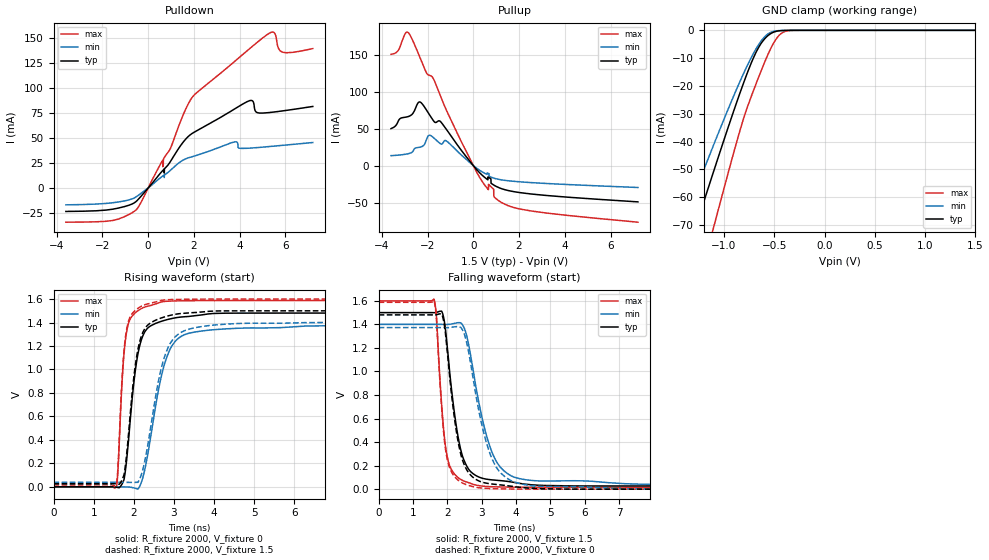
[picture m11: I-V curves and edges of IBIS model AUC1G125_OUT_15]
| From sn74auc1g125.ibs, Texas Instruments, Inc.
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[Model]   AUC1G125_OUT_15
Model_type  3-state
Enable   Active-Low
Vref =   0
Rref =   2000
Cref =   15p
Vmeas =   0.75
| variable   typ   min   max
C_comp   8.47pF   5.30pF   18.91pF
| C_pullup   7.46pF   4.00pF   14.06pF
| C_pulldown   10.53pF   5.76pF   20.41pF
| C_tri-state   8.47pF   5.30pF   18.91pF
[Temperature Range]   40   100   -40
| Ambient temperature   25   85   -40
[Voltage range]   1.5   1.4   1.6
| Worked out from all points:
|   slope of the pulldown table from 0 to 0.225 V, typ, clamps not added: 37 ohm
|   slope of the pullup table from 0 to 0.225 V, typ, clamps not added: 28.1 ohm
|   GND clamp passes 1 mA (typ) near -0.53 V on its own axis
|   rising waveform, R_fixture 2000, V_fixture 0: 20-80 % time 294ps typ, 469ps min, 169ps max; typ from 0 V to 1.48 V
|   falling waveform, R_fixture 2000, V_fixture 1.5: 20-80 % time 403ps typ, 622ps min, 244ps max; typ from 1.5 V to 0.027 V
|   rising waveform, R_fixture 2000, V_fixture 1.5: 20-80 % time 291ps typ, 461ps min, 167ps max; typ from 0.027 V to 1.5 V
|   falling waveform, R_fixture 2000, V_fixture 0: 20-80 % time 400ps typ, 617ps min, 242ps max; typ from 1.48 V to 0 V
[GND Clamp]
| AUC1G125_OUT_15A
|   Voltage   I(typ)   I(min)   I(max)
-3.6V     -338.8mA   -286.3mA   -409.7mA
-1.415V   -86.02mA   -70.29mA   -113.7mA
-1.265V   -68.97mA   -56.18mA   -93.1mA
-1.125V   -53.25mA   -43.26mA   -73.93mA
-1.085V   -48.8mA    -39.63mA   -68.47mA
-840mV    -22.47mA   -18.35mA   -35.96mA
-690mV    -8.595mA   -7.233mA   -20.12mA
-570mV    -2.132mA   -1.506mA   -9.318mA
-495mV    -520.9uA   -290.7uA   -3.905mA
-430mV    -104.6uA   -59.7uA    -1.117mA
-285mV    -1.435uA   -1.295uA   -9.372uA
1.5V      350.7pA    6.413nA    352.9pA
[Pulldown]
| AUC1G125_OUT_15A
|   Voltage   I(typ)   I(min)   I(max)
-3.6V     -23.47mA   -16.88mA   -34.23mA
-530mV    -13.56mA   -8.913mA   -21.94mA
630mV     17.27mA    11.79mA    27.62mA
655mV     17.88mA    12.18mA    21.8mA
1.92V     54.51mA    31.29mA    90.56mA
3.785V    79.13mA    46.19mA    126.7mA
4.44V     87.4mA     39.87mA    139.4mA
4.73V     75.86mA    40.35mA    145mA
5.195V    75.25mA    41.24mA    153.3mA
5.52V     76.05mA    41.91mA    155.3mA
5.885V    77.14mA    42.68mA    135.8mA
7.2V      81.56mA    45.48mA    139.5mA
[Pullup]
| AUC1G125_OUT_15A
|   Voltage   I(typ)   I(min)   I(max)
-3.6V     50.13mA    13.5mA     150.8mA
-2.81V    66.89mA    16.45mA    178.9mA
-2.355V   86.34mA    24.86mA    148.1mA
-1.89V    67.6mA     41.14mA    122.1mA
-1.415V   59mA       29.23mA    92.64mA
-1.175V   48.95mA    33.41mA    74.96mA
170mV     -6.178mA   -4.065mA   -10.23mA
890mV     -26.25mA   -16.87mA   -32.02mA
905mV     -26.53mA   -17.02mA   -41.95mA
1.12V     -29.9mA    -18.7mA    -47.79mA
2.525V    -38.43mA   -23mA      -61.43mA
7.2V      -49.13mA   -29.64mA   -76.65mA
[Ramp]
| AUC1G125_OUT_15A
| variable   typ   min   max
dV/dt_r   0.89/2.96E-10   0.84/4.79E-10   0.96/1.71E-10
dV/dt_f   0.89/4.06E-10   0.82/6.27E-10   0.96/2.46E-10
R_load = 2000
[Rising Waveform]
| AUC1G125_OUT_15A
R_fixture =   2000
C_fixture =   0
L_fixture =   0
V_fixture =   0
V_fixture_min = 0
V_fixture_max = 0
|   Time   V(typ)   V(min)   V(max)
0s        6.387nV    23.65nV    864.9pV
1.57ns    -3.297mV   8.561uV    4.787mV
1.735ns   43.44mV    -139.1uV   1.039V
1.855ns   343.3mV    -1.642mV   1.375V
2.015ns   925.7mV    -10.26mV   1.476V
2.165ns   1.225V     17.78mV    1.514V
2.73ns    1.415V     1.001V     1.578V
3.195ns   1.448V     1.285V     1.585V
4.585ns   1.48V      1.351V     1.587V
29.99ns   1.481V     1.373V     1.587V
[Falling Waveform]
| AUC1G125_OUT_15A
R_fixture =   2000
C_fixture =   0
L_fixture =   0
V_fixture =   1.5
V_fixture_min = 1.4
V_fixture_max = 1.6
|   Time   V(typ)   V(min)   V(max)
0s        1.5V       1.4V       1.6V
1.61ns    1.499V     1.4V       1.615V
1.68ns    1.502V     1.4V       1.474V
1.835ns   1.511V     1.4V       713.3mV
2.025ns   1.129V     1.399V     240mV
2.365ns   366.6mV    1.414V     87.16mV
2.89ns    106.6mV    777.3mV    31.27mV
3.465ns   74.44mV    217.1mV    19.05mV
4.455ns   36.93mV    73.69mV    16.52mV
29.99ns   27.18mV    38.78mV    16.4mV
[Rising Waveform]
| AUC1G125_OUT_15A
R_fixture =   2000
C_fixture =   0
L_fixture =   0
V_fixture =   1.5
V_fixture_min = 1.4
V_fixture_max = 1.6
|   Time   V(typ)   V(min)   V(max)
0s        27.17mV    38.78mV    16.4mV
1.555ns   25.42mV    38.78mV    17.78mV
1.605ns   22.9mV     38.78mV    164.5mV
1.74ns    86.89mV    38.68mV    1.09V
1.855ns   393.9mV    38.06mV    1.395V
2.16ns    1.252V     77.42mV    1.533V
2.72ns    1.443V     1.055V     1.591V
3.215ns   1.478V     1.323V     1.598V
4.635ns   1.5V       1.392V     1.6V
29.99ns   1.5V       1.4V       1.6V
[Falling Waveform]
| AUC1G125_OUT_15A
R_fixture =   2000
C_fixture =   0
L_fixture =   0
V_fixture =   0
V_fixture_min = 0
V_fixture_max = 0
|   Time   V(typ)   V(min)   V(max)
0s        1.481V     1.373V     1.587V
1.61ns    1.48V      1.373V     1.602V
1.68ns    1.482V     1.373V     1.456V
1.835ns   1.487V     1.373V     686.9mV
2.015ns   1.118V     1.372V     231.5mV
2.34ns    363mV      1.379V     69.94mV
2.825ns   84mV       808.6mV    16.01mV
3.425ns   39.65mV    186.8mV    3.231mV
4.49ns    6.775mV    27.7mV     65.64uV
29.99ns   3.474uV    -1.07uV    134.7nV
